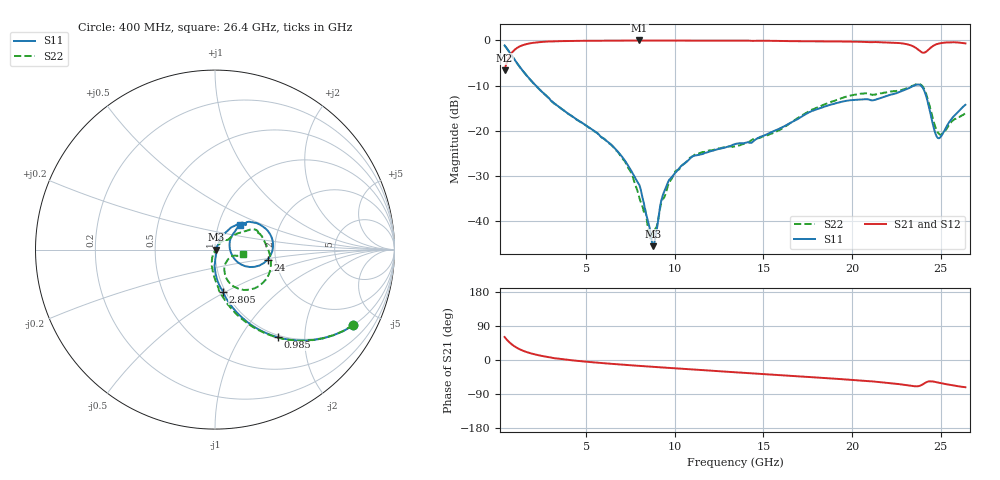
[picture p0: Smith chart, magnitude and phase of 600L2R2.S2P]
!  American Technical Ceramics  Date:  10/27/06
!  One Norden Lane
!  Huntington Station,  NY.  11746-2102
!  Tel:  (631) 622-4700  Fax:  (631) 622-4748
!  Part Number  600L2R2		Mounting Orientation: Vertical
!  Description: Ultra Low ESR Microwave capacitors
!  Application: Coupling, Bypass, Tuning, DC Block
!  Filters, Matching
# GHZ S DB R 50
! Freq  |S11|  S11 Ph  |S21|  S21 Ph  |S12|  S12 Ph  |S22|  S22 Ph
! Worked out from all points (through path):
!   401 points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, 400 MHz to 26.4 GHz, reference 50 ohm
!   highest |S21| = -0.02 dB at 8.005 GHz (marker M1); lowest = -6.6 dB at 400 MHz (marker M2)
!   group delay of S21, straight-line fit = 9.84 ps
!   lowest |S11| = -45.5 dB at 8.785 GHz (marker M3), VSWR 1.01, Z = 50.5 - j0.0951 ohm
!   |S11| at or under -10 dB: 2.16 GHz to 23.51 GHz (21.35 GHz wide, 166 % of centre); 23.89 GHz to end of sweep
!   |S22| runs from -43.9 to -1.1 dB; largest |S21 - S12| = 0.0042
!   S11 on the Smith chart (normalised r, x): 400 MHz: 0.99, -3.66; 985 MHz: 0.97, -1.48; 2.805 GHz: 0.97, -0.48; 24 GHz: 1.81, -0.22; 26.4 GHz: 1.27, +0.35
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0.4  -1.12 -28.7  -6.59 60.7  -6.60 60.6  -1.14 -28.7
0.985  -4.40 -54.2  -2.01 35.2  -2.02 35.2  -4.40 -54.5
1.7  -8.03 -69.0  -0.76 20.1  -0.77 20.1  -8.07 -70.4
2.805  -12.45 -79.6  -0.26 8.2  -0.27 8.2  -12.45 -83.4
4.755  -18.19 -89.3  -0.10 -3.4  -0.10 -3.4  -18.23 -95.7
6.9  -25.14 -88.8  -0.06 -11.8  -0.05 -11.7  -25.30 -106.9
7.55  -28.88 -83.4  -0.05 -14.0  -0.04 -14.0  -29.29 -111.8
8.005  -32.00 -75.9  -0.02 -15.6  -0.02 -15.6  -34.86 -105.0
8.59  -41.56 -53.4  -0.06 -17.6  -0.05 -17.5  -43.94 -50.9
8.785  -45.53 -10.2  -0.06 -18.1  -0.05 -18.0  -42.88 -15.7
9.11  -38.52 54.2  -0.06 -19.2  -0.05 -19.2  -38.66 33.0
9.63  -31.29 57.0  -0.06 -20.7  -0.05 -20.6  -32.00 50.0
10.8  -26.39 62.0  -0.05 -24.4  -0.05 -24.4  -26.16 53.9
13.4  -22.93 65.3  -0.06 -32.4  -0.05 -32.4  -23.43 46.0
17.755  -15.60 51.4  -0.20 -45.5  -0.19 -45.5  -15.31 33.6
22.11  -12.10 38.6  -0.47 -60.8  -0.46 -60.9  -11.39 16.8
23.345  -10.31 22.5  -1.13 -68.2  -1.12 -68.4  -10.20 -6.5
23.995  -10.49 -10.7  -2.72 -64.3  -2.70 -64.5  -10.21 -44.4
24.385  -15.45 -29.7  -1.82 -56.3  -1.82 -56.4  -14.58 -67.6
24.71  -20.62 -13.2  -0.95 -58.1  -0.94 -58.3  -19.24 -61.0
24.905  -21.66 8.2  -0.69 -60.0  -0.69 -60.3  -20.65 -45.8
26.4  -14.25 43.9  -0.67 -71.8  -0.66 -72.0  -16.06 -9.3
